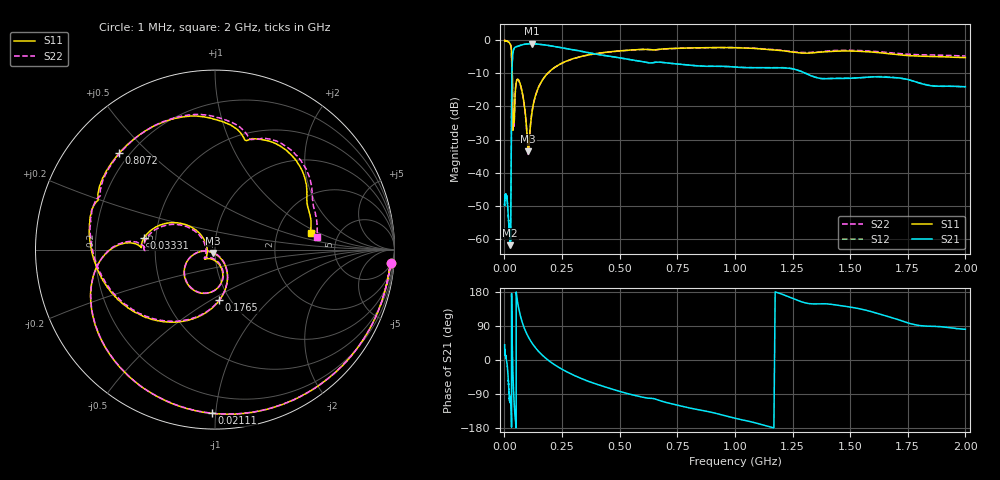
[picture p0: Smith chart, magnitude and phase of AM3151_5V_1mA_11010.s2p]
! Date/Time: Fri Jun 26 11:14:43 2020
! Network Analyzer:  Rev:
! Sweep from 1000000.0 to 2000000000.0, 1601 Points ! Power Supply: 0 V, 0 A
# HZ S DB R 50
!freq MagS11 AngS11 MagS21 AngS21 MagS12 AngS12 MagS22 AngS22
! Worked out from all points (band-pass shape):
!   1601 points, 1 MHz to 2 GHz, reference 50 ohm
!   highest |S21| = -1.15 dB at 119.6 MHz (marker M1); lowest = -61.8 dB at 25.17 MHz (marker M2)
!   |S21| within 3 dB of the highest: 36.55 MHz to 388.6 MHz (352.1 MHz wide, 166 % of centre)
!   lowest |S11| = -33.5 dB at 103.7 MHz (marker M3), VSWR 1.04, Z = 49 - j1.83 ohm
!   |S11| at or under -10 dB: 34.29 MHz to 188.8 MHz (154.6 MHz wide, 139 % of centre)
!   |S22| runs from -34.5 to -0.2 dB; largest |S21 - S12| = 0.0058
!   S11 on the Smith chart (normalised r, x): 1 MHz: 6, -25; 21.11 MHz: 0.09, -0.98; 33.31 MHz: 0.43, +0.07; 176.5 MHz: 0.89, -0.55; 807.2 MHz: 0.16, +0.41; 2 GHz: 3.13, +0.83
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1000000  -0.16 -4.3  -49.60 40.0  -49.86 36.0  -0.17 -4.3
3555161  -0.23 -14.4  -46.85 15.4  -46.82 15.4  -0.23 -14.4
1.263916e7  -0.41 -51.4  -48.63 -15.3  -48.71 -15.7  -0.41 -51.5
2.111241e7  -0.80 -91.2  -57.23 -94.7  -56.90 -93.5  -0.81 -91.4
2.516945e7  -1.19 -115.6  -61.82 -105.4  -61.00 -100.8  -1.20 -115.9
2.754699e7  -1.62 -134.1  -56.23 -104.5  -57.25 -105.5  -1.64 -134.6
3.146601e7  -5.53 176.7  -16.76 168.0  -16.76 167.9  -5.95 175.2
3.33119e7  -7.96 170.3  -8.33 70.2  -8.33 70.3  -8.12 173.0
3.680657e7  -26.44 161.9  -3.99 -29.9  -4.00 -29.9  -25.11 162.1
4.028332e7  -22.87 -134.6  -2.87 -88.4  -2.86 -88.4  -23.23 -139.1
4.493426e7  -19.31 -71.1  -2.27 -137.6  -2.27 -137.7  -19.57 -69.1
5.281102e7  -12.37 -96.7  -2.03 172.0  -2.02 172.0  -12.41 -96.2
6.857994e7  -13.27 -142.4  -1.66 118.9  -1.66 118.8  -13.34 -142.5
1.03679e8  -33.49 -118.1  -1.18 61.1  -1.18 61.1  -34.49 -115.0
1.195598e8  -21.86 -56.1  -1.15 45.0  -1.15 44.9  -21.84 -54.4
1.589914e8  -12.74 -75.9  -1.36 16.1  -1.36 16.0  -12.75 -75.8
1.765073e8  -10.95 -85.2  -1.52 6.3  -1.53 6.3  -10.97 -85.2
3.151132e8  -5.30 -136.5  -3.16 -44.0  -3.18 -44.0  -5.35 -137.6
5.652395e8  -2.98 170.3  -6.16 -93.4  -6.14 -93.4  -3.00 168.4
8.071763e8  -2.41 134.8  -7.63 -127.1  -7.60 -127.0  -2.42 132.4
1.125611e9  -2.77 90.6  -8.37 -171.9  -8.35 -171.9  -2.67 88.2
2e9  -5.32 9.9  -14.06 81.1  -14.21 80.5  -4.84 6.8
